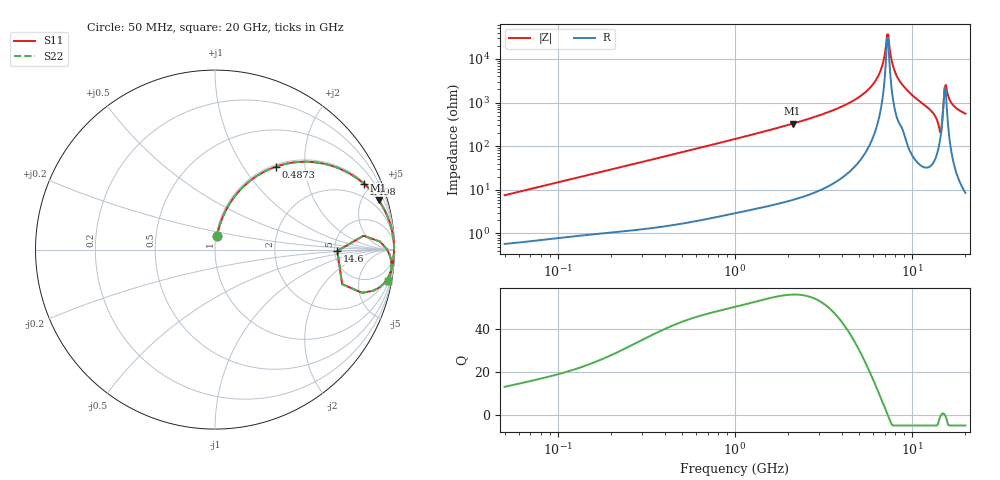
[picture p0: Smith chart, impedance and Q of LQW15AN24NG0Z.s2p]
!Murata Part Number: LQW15AN24NG0Z
!These Parameters are Measured in Series Mode Connection
!  o--[Z]--o
!Port1  Port2
!  o-------o
!Freq. Start=50[MHz] Stop=20[GHz], 401[Steps]
# Hz S RI R 50
!Freq.(Hz) S11(Real) S11(Imag) S21(Real) S21(Imag) S12(Real) S12(Imag) S22(Real) S22(Imag)
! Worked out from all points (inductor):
!   401 points, 50 MHz to 20 GHz, reference 50 ohm
!   read as one part in series: L = 23.7 nH near 51.52 MHz
!   highest Q = 56.1 at 2.115 GHz (marker M1), where L = 24.7 nH
!   self-resonance near 7.222 GHz
!   S11 on the Smith chart (normalised r, x): 50 MHz: 1.01, +0.15; 487.3 MHz: 1.03, +1.41; 1.498 GHz: 1.08, +4.47; 14.6 GHz: 5.28, -0.15; 20 GHz: 1, -11
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5e7  0.0112 0.0737  0.9888 -0.0737  0.9888 -0.0737  0.0112 0.0737
1.364002e8  0.0465 0.1894  0.9535 -0.1894  0.9535 -0.1894  0.0465 0.1894
3.721004e8  0.232 0.4094  0.768 -0.4094  0.768 -0.4094  0.232 0.4094
4.872511e8  0.3372 0.4613  0.6628 -0.4613  0.6628 -0.4613  0.3372 0.4613
1e9  0.6781 0.4574  0.3219 -0.4574  0.3219 -0.4574  0.6781 0.4574
1.498439e9  0.8286 0.3677  0.1714 -0.3677  0.1714 -0.3677  0.8286 0.3677
2.114743e9  0.9111 0.2758  0.0889 -0.2758  0.0889 -0.2758  0.9111 0.2758
2.728004e9  0.9495 0.2101  0.0505 -0.2101  0.0505 -0.2101  0.9495 0.2101
5.515528e9  0.9946 0.0549  0.00539 -0.0549  0.00539 -0.0549  0.9946 0.0549
6.406762e9  0.9971 0.0253  0.00291 -0.0253  0.00291 -0.0253  0.9971 0.0253
6.802353e9  0.9976 0.0135  0.00244 -0.0135  0.00244 -0.0135  0.9976 0.0135
7.114996e9  0.9977 0.00452  0.0023 -0.00452  0.0023 -0.00452  0.9977 0.00452
7.442007e9  0.9977 -0.0045  0.00235 0.0045  0.00235 0.0045  0.9977 -0.0045
7.901521e9  0.9972 -0.0167  0.00279 0.0167  0.00279 0.0167  0.9972 -0.0167
8.644534e9  0.9951 -0.035  0.00487 0.035  0.00487 0.035  0.9951 -0.035
1.276073e10  0.9698 -0.1462  0.0302 0.1462  0.0302 0.1462  0.9698 -0.1462
1.396067e10  0.8844 -0.2284  0.1156 0.2284  0.1156 0.2284  0.8844 -0.2284
1.460232e10  0.6818 -0.00759  0.3182 0.00759  0.3182 0.00759  0.6818 -0.00759
1.527346e10  0.9564 0.00435  0.0436 -0.00435  0.0436 -0.00435  0.9564 0.00435
1.573793e10  0.9786 -0.0485  0.0214 0.0485  0.0214 0.0485  0.9786 -0.0485
1.696185e10  0.9815 -0.1091  0.0185 0.1091  0.0185 0.1091  0.9815 -0.1091
2e10  0.9664 -0.1727  0.0336 0.1727  0.0336 0.1727  0.9664 -0.1727
